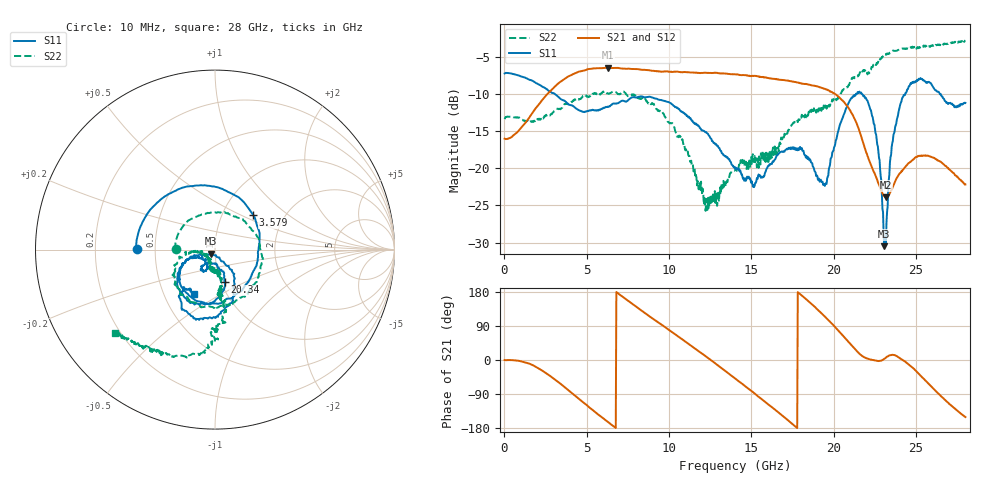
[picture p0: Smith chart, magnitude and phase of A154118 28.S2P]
!  2-Port S-parameters saved by WinCal
! VAR MeasName=S-Parameters (CALIBRATED_DATA) read from VNA (N5230A)
! VAR MeasDate=2015-9-10 14:36:28
! VAR NAME=A154118 28
! VAR FILENAME=A154118 28.S2P
! VAR DATE=2015-9-10 14:36:28
! VAR PHYS_PORTS=1,2
# Hz S DB R 50
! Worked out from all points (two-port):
!   801 points, 10 MHz to 28 GHz, reference 50 ohm
!   highest |S21| = -6.44 dB at 6.308 GHz (marker M1); lowest = -23.9 dB at 23.17 GHz (marker M2)
!   |S21| within 3 dB of the highest: 2.852 GHz to 19.65 GHz (16.8 GHz wide, 149 % of centre)
!   lowest |S11| = -30.5 dB at 23.07 GHz (marker M3), VSWR 1.06, Z = 48 - j2.1 ohm
!   |S11| at or under -10 dB: 3.072 GHz to 21.35 GHz (18.27 GHz wide, 150 % of centre); 21.72 GHz to 24.34 GHz (2.619 GHz wide, 11.4 % of centre); 26.5 GHz to end of sweep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
!   |S22| runs from -25.7 to -2.8 dB; largest |S21 - S12| = 0.0075
!   S11 on the Smith chart (normalised r, x): 10 MHz: 0.39, +0.00; 3.579 GHz: 1.40, +0.59; 20.34 GHz: 1.04, -0.39; 28 GHz: 0.70, -0.38
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1e7  -7.21 179.6  -16.00 -0.1  -16.03 -0.3  -13.36 179.8
1.794362e9  -8.30 114.0  -12.20 -15.3  -12.21 -15.1  -13.59 85.4
3.578725e9  -10.84 42.1  -8.05 -68.8  -8.05 -68.9  -11.59 -7.0
4.698325e9  -12.33 -0.5  -6.90 -108.7  -6.87 -109.0  -10.48 -50.8
6.30775e9  -11.73 -47.8  -6.44 -164.3  -6.41 -164.4  -9.94 -94.8
9.351662e9  -10.72 -120.9  -6.95 98.8  -6.89 98.6  -12.18 -156.4
1.229061e10  -15.23 -159.5  -7.12 7.8  -7.08 7.2  -25.23 -142.0
1.4005e10  -19.92 -155.9  -7.34 -48.5  -7.33 -49.0  -20.21 -106.2
1.585934e10  -20.47 -118.5  -7.77 -111.7  -7.70 -112.1  -19.14 -92.3
1.725884e10  -17.23 -117.2  -8.17 -160.3  -8.16 -161.1  -14.87 -78.7
1.869332e10  -19.30 -125.8  -8.83 146.4  -8.86 145.8  -11.89 -83.8
1.949804e10  -22.06 -88.8  -9.33 113.0  -9.33 112.8  -11.53 -83.3
2.033774e10  -14.42 -73.8  -10.44 74.9  -10.42 74.2  -10.28 -80.8
2.208711e10  -11.11 -138.6  -18.48 3.3  -18.56 2.2  -7.11 -91.7
2.264691e10  -16.81 -163.3  -21.57 -2.7  -21.68 -3.5  -5.89 -90.0
2.306676e10  -30.49 -132.9  -23.76 2.8  -23.82 2.4  -4.84 -96.4
2.317172e10  -30.33 -82.1  -23.91 6.0  -23.99 5.2  -4.71 -97.6
2.334666e10  -21.56 -54.4  -23.54 11.1  -23.58 10.6  -4.54 -100.7
2.387148e10  -13.10 -60.3  -21.12 9.1  -21.09 8.5  -4.11 -109.2
2.471118e10  -8.60 -88.3  -19.03 -17.6  -19.06 -18.2  -3.76 -116.8
2.583078e10  -8.44 -119.4  -18.37 -65.8  -18.39 -66.5  -3.63 -124.3
2.8e10  -11.18 -115.7  -22.18 -150.6  -22.27 -150.9  -2.76 -140.2
